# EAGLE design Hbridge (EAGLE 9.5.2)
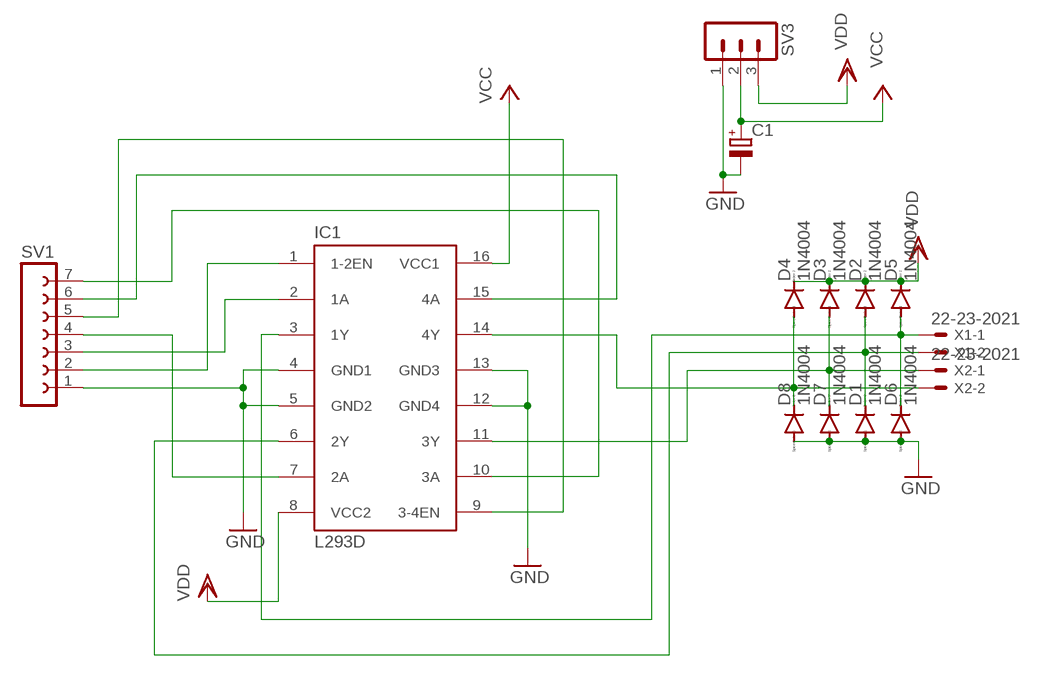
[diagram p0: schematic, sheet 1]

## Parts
C1  CPOL-EUE2-5  [E2-5]
D1  1N4004  [DO41-10]
D2  1N4004  [DO41-10]
D3  1N4004  [DO41-10]
D4  1N4004  [DO41-10]
D5  1N4004  [DO41-10]
D6  1N4004  [DO41-10]
D7  1N4004  [DO41-10]
D8  1N4004  [DO41-10]
IC1  L293D  [DIL16]
SV1  FE07-1  [FE07]
SV3  MA03-1  [MA03-1]
X1  22-23-2021  [22-23-2021]
X2  22-23-2021  [22-23-2021]

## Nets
GND: C1.- D1.A D6.A D7.A D8.A IC1.4(GND1) IC1.5(GND2) IC1.12(GND4) IC1.13(GND3) SV1.1 SV3.1
N$1: IC1.2(1A) SV1.3
N$2: IC1.7(2A) SV1.4
N$3: IC1.1(1-2EN) SV1.2
N$4: IC1.10(3A) SV1.7
N$5: IC1.15(4A) SV1.6
N$6: IC1.9(3-4EN) SV1.5
N$7: D5.A D6.C IC1.3(1Y) X1.1
N$8: D1.C D2.A IC1.6(2Y) X1.2
N$9: D3.A D7.C IC1.11(3Y) X2.1
N$10: D4.A D8.C IC1.14(4Y) X2.2
VCC: C1.+ IC1.16(VCC1) SV3.2
VDD: D2.C D3.C D4.C D5.C IC1.8(VCC2) SV3.3

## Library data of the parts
C1 = rcl-mod:CPOL-EU: POLARIZED CAPACITOR, European symbol; SPICEPREFIX: C
D1-D8 = diode-mod:1N4004: DIODE
IC1 = st-microelectronics-mod:L293D: PUSH-PULL 4 CHANNEL DRIVER; MPN: L293D; OC_FARNELL: 9589619; OC_NEWARK: 56P8249
SV1 = con-lsta:FE07-1: FEMALE HEADER; OC_FARNELL: unknown; OC_NEWARK: unknown
SV3 = con-lstb:MA03-1: PIN HEADER; OC_FARNELL: unknown; OC_NEWARK: unknown
X1 X2 = con-molex:22-23-2021: .100" (2.54mm) Center Header - 2 Pin; MF: MOLEX; MPN: 22-23-2021; OC_FARNELL: 1462926; OC_NEWARK: 25C3832

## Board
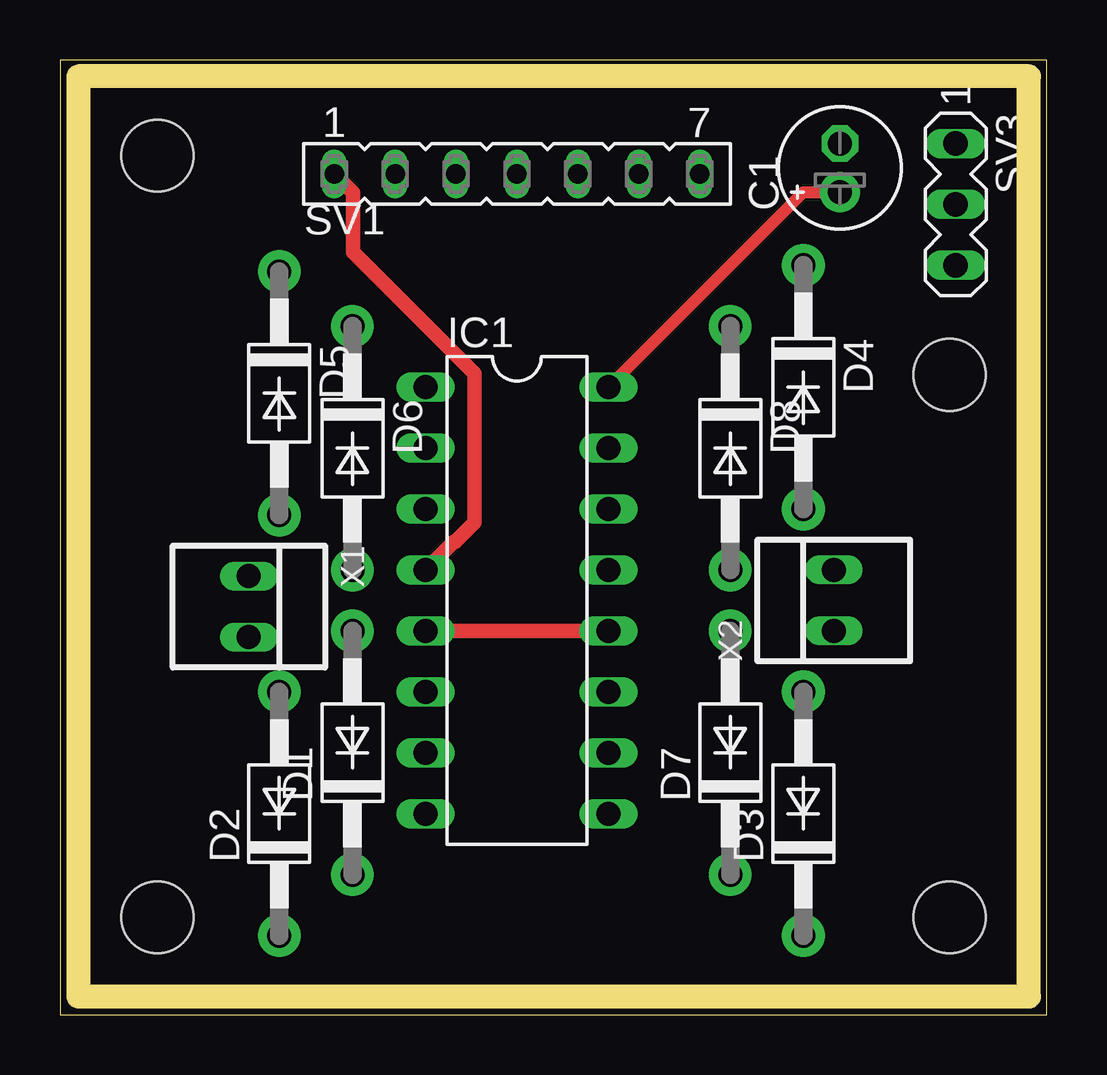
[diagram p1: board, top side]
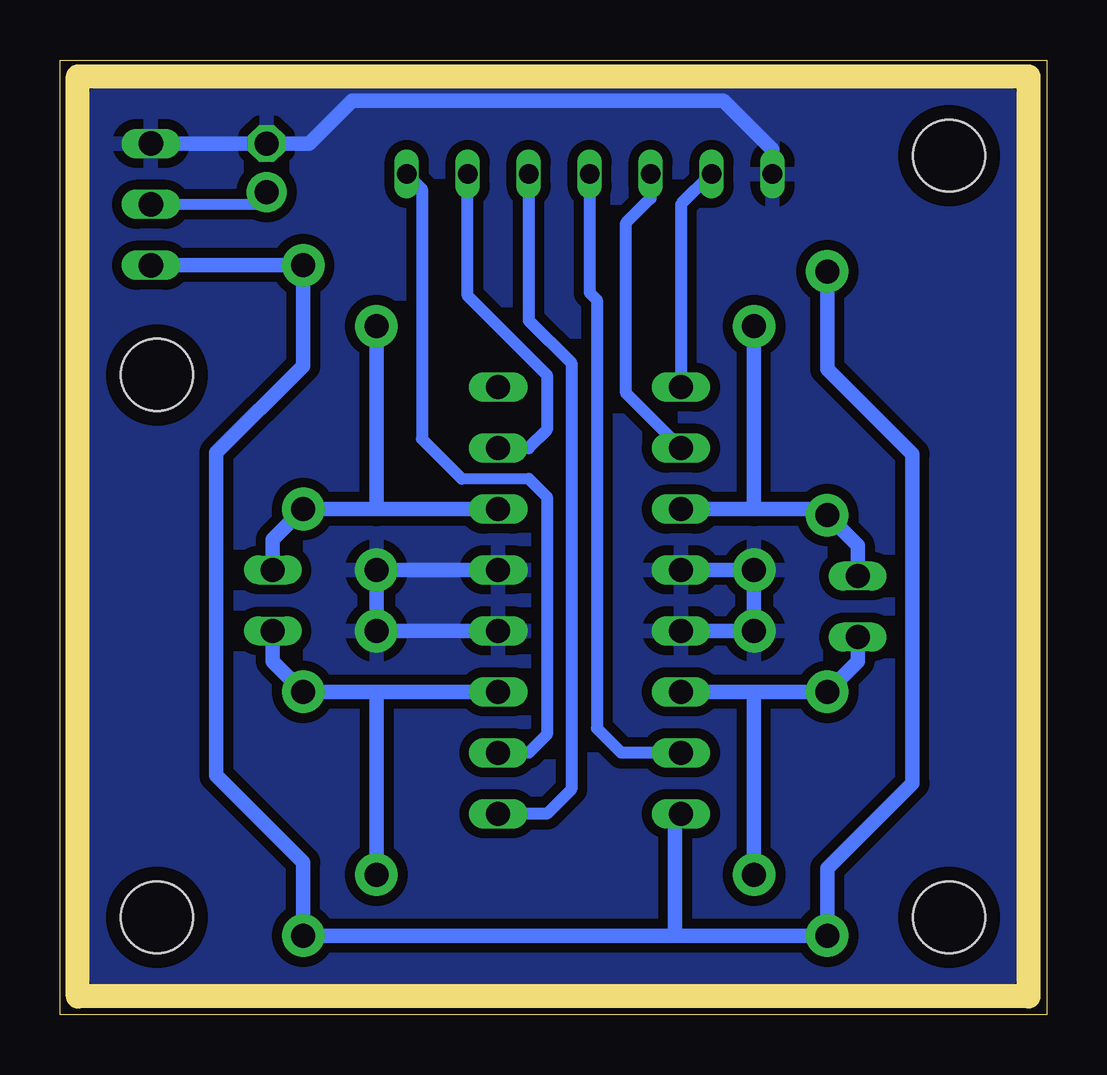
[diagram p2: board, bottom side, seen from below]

Size 41.13 x 39.8 mm. Coordinates in mm from the lower left corner, seen from the top.
Outline: 0,0 41.13,0 41.13,39.8 0,39.8 0,0
Copper layers (1*16): Top 0.035mm / dielectric 1.5mm / Bottom 0.035mm
Design rules "default *": minimum track width 6mil, minimum drill 0.35mm, track to track 16mil, track to pad 16mil, pad to pad 16mil, via to via 16mil, smd to smd 16mil, copper to edge 24mil, drill to drill 6mil, minimum pad ring 4mil, minimum via ring 4mil, stop-mask expansion 4mil, vias tented up to drill 0mil, thermal gap 16mil
Holes 3 mm at 4.06,4.06 37.08,4.06 4.06,35.81 37.08,26.67
Milling: 4 lines

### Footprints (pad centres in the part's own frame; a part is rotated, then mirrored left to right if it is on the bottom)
E2-5 = drill 1 pad 1.676: + -1.016,0 | drill 1 pad 1.524 octagon: - 1.016,0
DO41-10 = drill 1 pad 1.778: A 5.08,0; C -5.08,0
DIL16 = drill 1 pad 1.219 long: 1 -8.89,-3.81; 2 -6.35,-3.81; 3 -3.81,-3.81; 4 -1.27,-3.81; 5 1.27,-3.81; 6 3.81,-3.81; 7 6.35,-3.81; 8 8.89,-3.81; 9 8.89,3.81; 10 6.35,3.81; 11 3.81,3.81; 12 1.27,3.81; 13 -1.27,3.81; 14 -3.81,3.81; 15 -6.35,3.81; 16 -8.89,3.81
FE07 = drill 0.813 long: 1 -7.62,0; 2 -5.08,0; 3 -2.54,0; 4 0,0; 5 2.54,0; 6 5.08,0; 7 7.62,0
MA03-1 = drill 1.016 long: 1 -2.54,0; 2 0,0; 3 2.54,0
22-23-2021 = drill 1 long: 1 -1.27,0; 2 1.27,0

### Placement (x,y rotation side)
C1  32.51,35.31 90 top
D1  12.19,10.92 90 top
D2  9.14,8.38 90 top
D3  30.99,8.38 90 top
D4  30.99,26.16 270 top
D5  9.14,25.91 270 top
D6  12.19,23.62 270 top
D7  27.94,10.92 90 top
D8  27.94,23.62 270 top
IC1  19.05,17.27 270 top
SV1  19.05,35.05 0 top
SV3  37.34,33.78 270 top
X1  7.87,17.02 270 top
X2  32.26,17.27 90 top

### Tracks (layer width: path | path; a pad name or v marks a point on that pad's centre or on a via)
GND
  Top 0.61: SV1.1 12.22,34.27 12.22,31.79 17.27,26.73 17.27,20.51 16.47,19.71 16.41,19.71 IC1.4 | IC1.5 IC1.12
  Bottom 0.61: IC1.12 D7.A D8.A IC1.13 | IC1.5 D1.A D6.A IC1.4 | SV1.1 11.43,36.07 13.46,38.1 28.96,38.1 30.73,36.32 C1.- SV3.1
  pour Bottom (isolate 0.406): 1.52,38.35 39.62,38.35 39.62,1.52 1.52,1.52
N$1
  Bottom 0.508: IC1.2 17.53,25.91 17.53,33.02 16.51,34.04 SV1.3
N$2
  Bottom 0.508: IC1.7 17.73,10.92 18.75,11.94 18.75,29.8 19.05,30.11 SV1.4
N$3
  Bottom 0.508: SV1.2 15.24,33.78 IC1.1
N$4
  Bottom 0.457: 24.38,22.35 21.59,22.35
  Bottom 0.508: SV1.7 26.04,34.42 26.04,24 24.38,22.35 | 21.59,22.35 20.83,21.59 20.83,11.68 21.59,10.92 IC1.10
N$5
  Bottom 0.508: IC1.15 21.59,23.62 20.83,24.38 20.83,26.67 24.13,29.97 SV1.6
N$6
  Bottom 0.508: SV1.5 21.59,28.96 19.81,27.18 19.81,9.4 20.83,8.38 IC1.9
N$7
  Bottom 0.61: 12.19,21.08 9.4,21.08 D5.A 7.87,19.56 X1.1 | 12.19,21.08 IC1.3 | 12.19,21.08 D6.C
N$8
  Bottom 0.61: 12.19,13.46 D2.A 7.87,14.73 X1.2 | 12.19,13.46 IC1.6 | D1.C 12.19,13.46
N$9
  Bottom 0.61: IC1.11 27.94,13.46 | 27.94,13.46 D7.C | 27.94,13.46 D3.A 32.26,14.73 X2.1
N$10
  Bottom 0.61: 27.94,21.08 D8.C | IC1.14 27.94,21.08 | 27.94,21.08 D4.A 32.26,19.81 X2.2
VCC
  Top 0.508: IC1.16 30.99,34.29 C1.+
  Bottom 0.457: SV3.2 32.51,33.78 C1.+
VDD
  Bottom 0.61: IC1.8 15.49,8.13 15.49,3.3 | 15.49,3.3 D2.C 9.14,6.1 5.59,9.65 5.59,23.37 9.14,26.92 D5.C | 15.49,3.3 D3.C 30.99,6.35 34.61,9.97 34.61,23.43 30.99,27.05 D4.C SV3.3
